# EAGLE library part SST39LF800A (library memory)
8 Mbit (x16) Multi-Purpose Flash Source: http://www.sst.com/dotAsset/40687.pdf
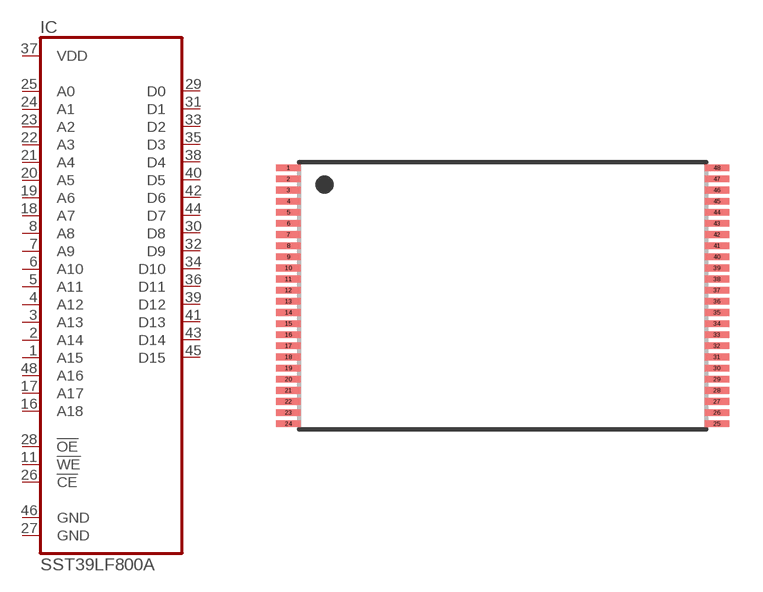
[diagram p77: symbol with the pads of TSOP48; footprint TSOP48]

Designator prefix IC

## SST39LF800A  [TSOP48]
1  A15  in
2  A14  in
3  A13  in
4  A12  in
5  A11  in
6  A10  in
7  A9  in
8  A8  in
11  !WE  in
16  A18  in
17  A17  in
18  A7  in
19  A6  in
20  A5  in
21  A4  in
22  A3  in
23  A2  in
24  A1  in
25  A0  in
26  !CE  in
27  GND  pwr
28  !OE  in
29  D0
30  D8
31  D1
32  D9
33  D2
34  D10
35  D3
36  D11
37  VDD  pwr
38  D4
39  D12
40  D5
41  D13
42  D6
43  D14
44  D7
45  D15
46  GND  pwr
48  A16  in

## Footprint TSOP48 (pad centres in mm)
48-Lead Thin Small Outline Package (TSOP) 12mm x 20mm SST Package Code: EK Source: http://www.sst.com/dotAsset/40687.pdf
smd 1.1 x 0.3: 1 -9.625,5.75; 2 -9.625,5.25; 3 -9.625,4.75; 4 -9.625,4.25; 5 -9.625,3.75; 6 -9.625,3.25; 7 -9.625,2.75; 8 -9.625,2.25; 9 -9.625,1.75; 10 -9.625,1.25; 11 -9.625,0.75; 12 -9.625,0.25; 13 -9.625,-0.25; 14 -9.625,-0.75; 15 -9.625,-1.25; 16 -9.625,-1.75; 17 -9.625,-2.25; 18 -9.625,-2.75; 19 -9.625,-3.25; 20 -9.625,-3.75; 21 -9.625,-4.25; 22 -9.625,-4.75; 23 -9.625,-5.25; 24 -9.625,-5.75; 25 9.625,-5.75; 26 9.625,-5.25; 27 9.625,-4.75; 28 9.625,-4.25; 29 9.625,-3.75; 30 9.625,-3.25; 31 9.625,-2.75; 32 9.625,-2.25; 33 9.625,-1.75; 34 9.625,-1.25; 35 9.625,-0.75; 36 9.625,-0.25; 37 9.625,0.25; 38 9.625,0.75; 39 9.625,1.25; 40 9.625,1.75; 41 9.625,2.25; 42 9.625,2.75; 43 9.625,3.25; 44 9.625,3.75; 45 9.625,4.25; 46 9.625,4.75; 47 9.625,5.25; 48 9.625,5.75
